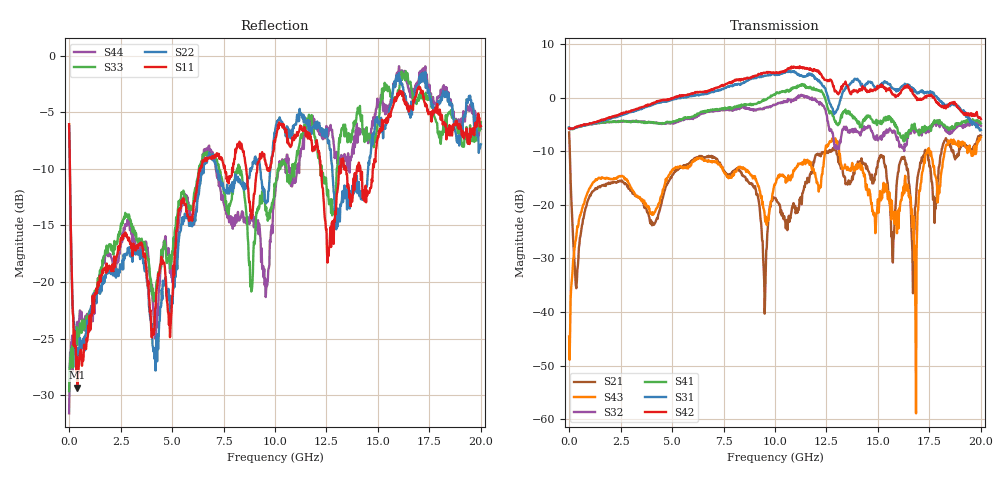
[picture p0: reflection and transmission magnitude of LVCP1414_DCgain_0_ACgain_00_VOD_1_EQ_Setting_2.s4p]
!Agilent Technologies,N5230A,MY46400459,A.07.50.48
!Agilent N5230A: A.07.50.48
!Date: Tuesday, April 17, 2012 18:26:27
!Correction: S11(Full 4 Port(1,2,3,4))
!S12(Full 4 Port(1,2,3,4))
!S13(Full 4 Port(1,2,3,4))
!S14(Full 4 Port(1,2,3,4))
!S21(Full 4 Port(1,2,3,4))
!S22(Full 4 Port(1,2,3,4))
!S23(Full 4 Port(1,2,3,4))
!S24(Full 4 Port(1,2,3,4))
!S31(Full 4 Port(1,2,3,4))
!S32(Full 4 Port(1,2,3,4))
!S33(Full 4 Port(1,2,3,4))
!S34(Full 4 Port(1,2,3,4))
!S41(Full 4 Port(1,2,3,4))
!S42(Full 4 Port(1,2,3,4))
!S43(Full 4 Port(1,2,3,4))
!S44(Full 4 Port(1,2,3,4))
!S4P File: Measurements: <S11,S12,S13,S14>,
!<S21,S22,S23,S24>,
!<S31,S32,S33,S34>,
!<S41,S42,S43,S44>:
# Hz S  dB  R 50
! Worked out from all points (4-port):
!   801 points, 300 kHz to 20 GHz, reference 50 ohm
!   strongest paths, dB at 300 kHz, 5 GHz, 10 GHz, 15 GHz, 20 GHz:
!     S42: -5.8, -0.1, 4.5, 2.0, -4.0
!     S31: -5.6, -0.4, 4.2, 1.8, -6.0
!     S41: -5.6, -4.5, 0.5, -4.4, -4.8
!     S32: -5.7, -4.7, -1.4, -8.0, -5.3
!     S43: -44.6, -13.5, -16.3, -19.0, -7.4
!     S21: -6.5, -14.5, -18.8, -11.9, -7.1
!   lowest |S11| = -29.3 dB at 400.3 MHz (marker M1), VSWR 1.07, Z = 53.1 + j1.63 ohm
!   |S11| at or under -10 dB: 37.57 MHz to 6.367 GHz (6.329 GHz wide, 198 % of centre); 12.21 GHz to 13.12 GHz (902 MHz wide, 7.12 % of centre); 14.15 GHz to 14.75 GHz (602.9 MHz wide, 4.17 % of centre)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
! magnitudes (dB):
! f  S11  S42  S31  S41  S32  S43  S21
! 300 kHz  -6.1  -5.8  -5.6  -5.6  -5.7  -44.6  -6.5
! 400.3 MHz  -29.3  -5.4  -5.4  -5.5  -5.5  -24.0  -32.2
! 9.95 GHz  -8.2  4.6  4.3  0.6  -1.4  -16.7  -18.7
! 12.88 GHz  -14.5  1.6  -3.1  -4.1  -8.7  -8.2  -9.7
! 16.8 GHz  -3.7  0.4  1.4  -5.5  -6.0  -32.2  -20.5
! 17.4 GHz  -4.9  0.3  1.1  -5.9  -5.9  -10.2  -10.3
! 20 GHz  -6.2  -4.0  -6.0  -4.8  -5.3  -7.4  -7.1
